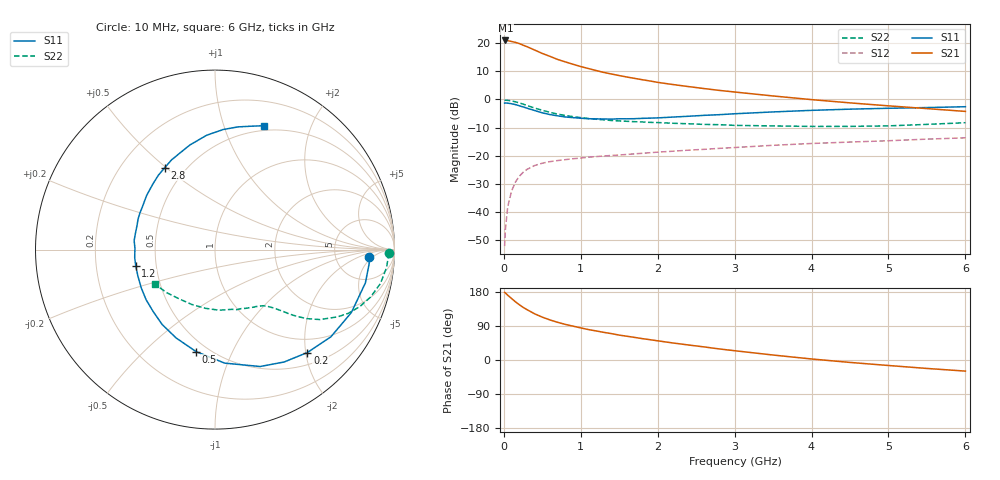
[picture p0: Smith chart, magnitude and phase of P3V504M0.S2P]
! SIEMENS Small Signal Semiconductors
! BFP181
! Si NPN RF Bipolar Junction Transistor in SOT143
! VCE = 0.5 V  IC = 4 mA
! Common Emitter S-Parameters:  March  1996
# GHz  S  MA  R  50
!  f  S11  S21  S12  S22
! GHz  MAG  ANG  MAG  ANG  MAG  ANG  MAG  ANG
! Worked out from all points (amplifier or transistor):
!   36 points, 10 MHz to 6 GHz, reference 50 ohm
!   highest |S21| = 20.9 dB at 20 MHz (marker M1)
!   |S21| within 3 dB of that: start of sweep to 367.5 MHz
!   unconditionally stable (mu >= 1): 1.169 GHz to end of sweep
!   at 250 MHz: K = 0.27, MSG = 22.5 dB, |S12| = -25.9 dB
!   at 1.4 GHz: K = 1.14, MAG = 12.2 dB, |S12| = -19.9 dB
!   at 6 GHz: K = 1.41, MAG = 0.9 dB, |S12| = -13.6 dB
!   S11 on the Smith chart (normalised r, x): 10 MHz: 12, -4; 200 MHz: 0.72, -2.03; 500 MHz: 0.43, -0.73; 1.2 GHz: 0.38, -0.09; 2.8 GHz: 0.39, +0.49; 6 GHz: 0.45, +1.37
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0.01  0.8599 -2.8  11.03 178.4  0.0025 84.6  0.9699 -1.1
0.02  0.8626 -5.2  11.07 176.9  0.0049 87.0  0.9663 -2.4
0.05  0.8582 -12.5  10.99 171.0  0.0124 84.6  0.961 -6.0
0.1  0.8367 -24.8  10.62 162.3  0.0236 75.1  0.9408 -11.6
0.15  0.8082 -36.9  10.26 153.7  0.0341 68.9  0.906 -17.0
0.2  0.7707 -48.1  9.757 146.1  0.0432 63.6  0.8669 -21.5
0.25  0.7351 -58.4  9.136 138.9  0.0508 58.5  0.8237 -25.5
0.3  0.6982 -68.9  8.604 133.0  0.0573 54.2  0.7798 -28.7
0.4  0.6349 -85.1  7.496 121.9  0.0672 47.5  0.7025 -33.7
0.5  0.5776 -100.6  6.513 113.1  0.0738 42.3  0.6407 -36.9
0.6  0.538 -113.7  5.785 105.7  0.0788 38.8  0.5887 -39.2
0.7  0.5107 -125.2  5.096 99.4  0.0824 36.4  0.5476 -40.9
0.9  0.4748 -143.9  4.189 89.3  0.0887 33.2  0.4944 -43.1
1.1  0.4543 -160.9  3.52 80.3  0.0944 31.1  0.458 -45.1
1.2  0.4509 -168.1  3.244 76.7  0.0967 30.1  0.4444 -46.1
1.6  0.4525 168.4  2.49 62.7  0.1057 28.8  0.4085 -50.1
2.2  0.4858 141.7  1.831 44.9  0.1206 26.8  0.377 -59.0
2.8  0.5354 121.5  1.443 29.2  0.1354 24.4  0.3559 -70.0
3.5  0.599 103.6  1.149 13.1  0.1535 21.0  0.3385 -86.1
4.5  0.6707 86.1  0.867 -6.4  0.1752 14.2  0.3319 -112.7
5.5  0.7158 73.8  0.686 -22.3  0.1974 8.6  0.3603 -138.2
6  0.7412 68.6  0.612 -29.3  0.2081 4.9  0.3859 -149.9
